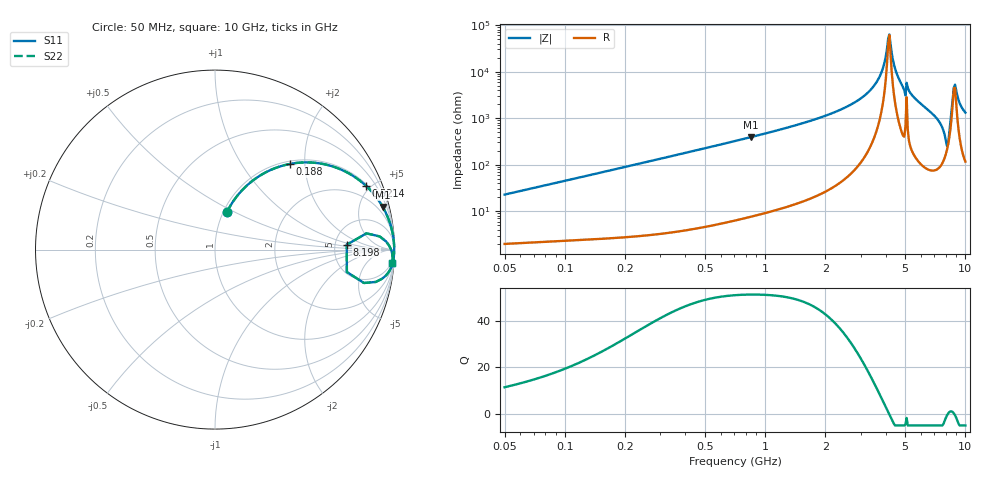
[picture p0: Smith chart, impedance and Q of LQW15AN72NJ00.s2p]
!Murata Part Number: LQW15AN72NJ00
!These Parameters are Measured in Series Mode Connection
!  o--[Z]--o
!Port1  Port2
!  o-------o
!Freq. Start=50[MHz] Stop=10[GHz], 401[Steps]
# Hz S RI R 50
!Freq.(Hz)	S 11(Real)	S 11(Imag)	S 21(Real)	S 21(Imag)	S 12(Real)	S 12(Imag)	S 22(Real)	S 22(Imag)
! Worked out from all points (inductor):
!   401 points, 50 MHz to 10 GHz, reference 50 ohm
!   read as one part in series: L = 72 nH near 51.34 MHz
!   highest Q = 51.4 at 851.2 MHz (marker M1), where L = 73.3 nH
!   self-resonance near 4.117 GHz
!   S11 on the Smith chart (normalised r, x): 50 MHz: 1.04, +0.45; 188 MHz: 1.05, +1.68; 521.4 MHz: 1.10, +4.70; 8.198 GHz: 6.44, +0.77; 10 GHz: 3, -26
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5e7  0.0658 0.208  0.9342 -0.208  0.9342 -0.208  0.0658 0.208
1.214486e8  0.2392 0.4049  0.7608 -0.4049  0.7608 -0.4049  0.2392 0.4049
1.880302e8  0.4177 0.4774  0.5823 -0.4774  0.5823 -0.4774  0.4177 0.4774
2.949953e8  0.6328 0.47  0.3672 -0.47  0.3672 -0.47  0.6328 0.47
5.214057e8  0.842 0.3548  0.158 -0.3548  0.158 -0.3548  0.842 0.3548
7.071068e8  0.9077 0.2798  0.0923 -0.2798  0.0923 -0.2798  0.9077 0.2798
8.511793e8  0.9349 0.2371  0.0651 -0.2371  0.0651 -0.2371  0.9349 0.2371
1.717543e9  0.9856 0.109  0.0144 -0.109  0.0144 -0.109  0.9856 0.109
2.555552e9  0.9951 0.0565  0.00492 -0.0565  0.00492 -0.0565  0.9951 0.0565
3.286879e9  0.9977 0.0271  0.00227 -0.0271  0.00227 -0.0271  0.9977 0.0271
3.752403e9  0.9984 0.012  0.00165 -0.012  0.00165 -0.012  0.9984 0.012
4.062795e9  0.9985 0.00273  0.00153 -0.00273  0.00153 -0.00273  0.9985 0.00273
4.171863e9  0.9985 -0.000406  0.00154 0.000406  0.00154 0.000406  0.9985 -0.000406
4.516952e9  0.9983 -0.0102  0.00171 0.0102  0.00171 0.0102  0.9983 -0.0102
4.890587e9  0.9975 -0.0218  0.00249 0.0218  0.00249 0.0218  0.9975 -0.0218
6.993273e9  0.9866 -0.0866  0.0134 0.0866  0.0134 0.0866  0.9866 -0.0866
7.775012e9  0.931 -0.1624  0.069 0.1624  0.069 0.1624  0.931 -0.1624
7.983737e9  0.8298 -0.186  0.1702 0.186  0.1702 0.186  0.8298 -0.186
8.198065e9  0.7342 0.0275  0.2658 -0.0275  0.2658 -0.0275  0.7342 0.0275
8.644138e9  0.9701 0.0224  0.0299 -0.0224  0.0299 -0.0224  0.9701 0.0224
8.876195e9  0.9839 -0.00949  0.0161 0.00949  0.0161 0.00949  0.9839 -0.00949
1e10  0.9877 -0.0744  0.0123 0.0744  0.0123 0.0744  0.9877 -0.0744
